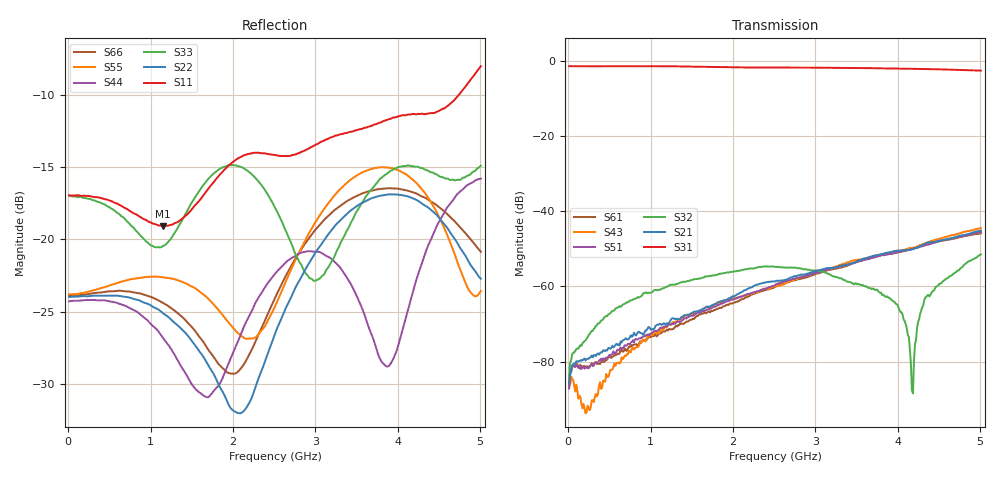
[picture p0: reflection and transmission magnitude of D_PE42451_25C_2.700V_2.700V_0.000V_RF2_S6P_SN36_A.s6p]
! Device ID: PE42451
! Serial: 36
! Insertion: A
! Temp: 25C
! VDD: 2.700
! Control_Hi: 100.000
! Control_Lo: 0.000
! Logic State: RF2
! Port 1: RFC
! Port 2: RF1
! Port 3: RF2
! Port 4: RF3
! Port 5: RF4
! Port 6: RF5
! V1 = 0.00
! V2 = 2.70
! V3 = 0.00
! V4 = 0.00
! IDD: 1.086280e-05
#  Hz  S  RI  R  50
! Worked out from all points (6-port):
!   401 points, 10 MHz to 5.01 GHz, reference 50 ohm
!   strongest paths, dB at 10 MHz, 1.26 GHz, 2.51 GHz, 3.76 GHz, 5.01 GHz:
!     S31: -1.4, -1.5, -1.8, -2.0, -2.6
!     S21: -85.9, -68.5, -58.7, -51.6, -45.2
!     S32: -83.9, -59.6, -54.8, -61.2, -51.5
!     S51: -87.1, -69.9, -59.6, -52.0, -45.5
!     S43: -84.5, -69.6, -59.9, -51.7, -44.5
!     S61: -86.7, -71.3, -60.1, -51.8, -45.9
!   lowest |S11| = -19.1 dB at 1.147 GHz (marker M1), VSWR 1.25, Z = 57.8 - j9.16 ohm
!   |S11| at or under -10 dB: start of sweep to 4.741 GHz
